VAR_GLOBAL
	(* These global connection and namespace settings need to be adapted to the runtime environment *)
	sOpcUaServerUrl : STRING(MAX_STRING_LENGTH) := 'opc.tcp://localhost:4840';
	sNamespaceUri : STRING(MAX_STRING_LENGTH) := 'urn:BeckhoffAutomation:Ua:PLC1'; // TF6100 setup version 4.x default
END_VAR
